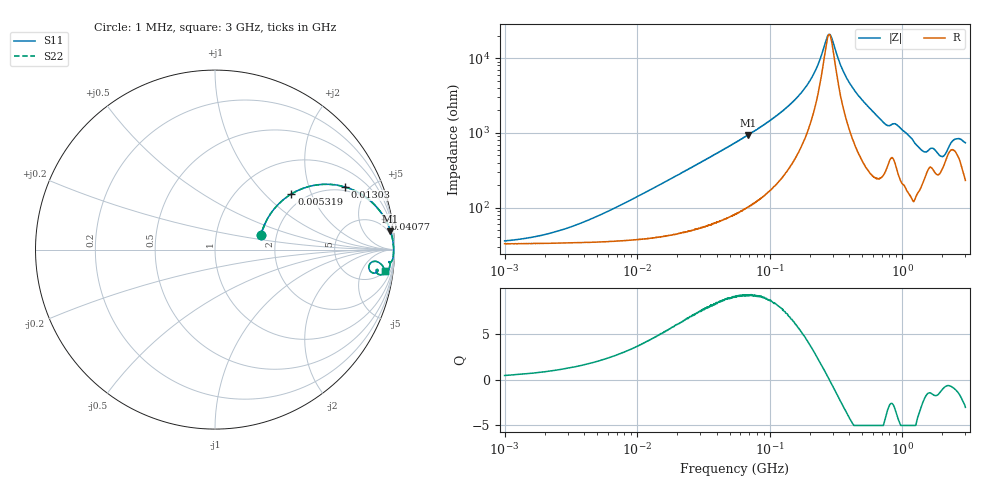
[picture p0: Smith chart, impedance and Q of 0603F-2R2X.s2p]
!s-Parameter Generated by FASTRON Sdn. Bhd.
!FASTRON P/N : 0603F-2R2X
!Keysight Technologies: E4991B_MY54100416_A.01.15
!Date: Wed Jun 19 15:55:30 2024
!Version  :Rev00  Wed Jun 19 15:55:30 2024
!Data & Calibration Information:
!Freq  S11  S21  S12  S22
!PortZ  Port1:50+j0  Port2:50+j0
!When reading reference impedance value at option line is always used.
! Remarks : This data is being provided solely for informational purposes.
# Hz S dB R 50
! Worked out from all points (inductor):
!   1601 points, 1 MHz to 3 GHz, reference 50 ohm
!   read as one part in series: L = 2.15 uH near 8.058 MHz
!   highest Q = 9.18 at 68.26 MHz (marker M1), where L = 2.18 uH
!   self-resonance near 281.3 MHz
!   S11 on the Smith chart (normalised r, x): 1 MHz: 1.66, +0.29; 5.319 MHz: 1.69, +1.46; 13.03 MHz: 1.79, +3.51; 40.77 MHz: 2, +11; 3 GHz: 6, -14
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1000000  -11.40 17.5  -2.53 -6.2  -2.53 -6.2  -11.40 17.5
3804036  -7.23 35.6  -3.17 -21.4  -3.17 -21.4  -7.23 35.6
5319234  -5.56 36.1  -3.71 -28.4  -3.71 -28.4  -5.56 36.1
1.302723e7  -1.91 25.8  -7.00 -51.5  -7.00 -51.5  -1.91 25.8
1.447069e7  -1.64 24.1  -7.59 -54.2  -7.59 -54.2  -1.64 24.1
4.07701e7  -0.32 10.1  -15.10 -73.1  -15.10 -73.1  -0.32 10.1
5.504702e7  -0.20 7.5  -17.60 -76.2  -17.60 -76.2  -0.20 7.5
6.826239e7  -0.15 6.0  -19.60 -77.8  -19.60 -77.8  -0.15 6.0
1.403209e8  -0.06 2.4  -27.50 -79.3  -27.50 -79.3  -0.06 2.4
2.083556e8  -0.05 1.0  -34.90 -72.6  -34.90 -72.6  -0.05 1.0
2.702786e8  -0.04 0.1  -45.50 -26.0  -45.50 -26.0  -0.04 0.1
2.841474e8  -0.04 -0.0  -46.40 5.7  -46.40 5.7  -0.04 -0.0
3.50605e8  -0.04 -0.7  -37.40 68.6  -37.40 68.6  -0.04 -0.7
4.135554e8  -0.05 -1.3  -32.70 76.3  -32.70 76.3  -0.05 -1.3
5.840965e8  -0.07 -2.8  -26.30 79.4  -26.30 79.4  -0.07 -2.8
7.925923e8  -0.24 -4.2  -22.20 67.1  -22.20 67.1  -0.24 -4.2
9.117997e8  -0.19 -4.2  -22.40 71.2  -22.40 71.2  -0.19 -4.2
1.452135e9  -0.70 -8.6  -15.70 57.7  -15.70 57.7  -0.70 -8.6
1.687342e9  -0.78 -7.1  -16.70 50.7  -16.70 50.7  -0.78 -7.1
1.990301e9  -1.19 -7.8  -14.90 41.2  -14.90 41.2  -1.19 -7.8
2.468121e9  -0.76 -4.5  -19.00 39.8  -19.00 39.8  -0.76 -4.5
3e9  -0.43 -7.0  -17.80 64.7  -17.80 64.7  -0.43 -7.0
